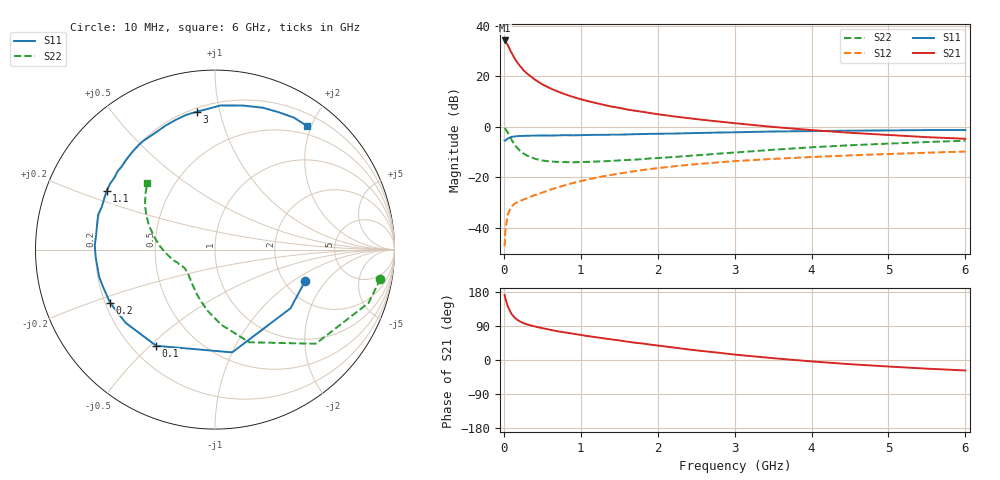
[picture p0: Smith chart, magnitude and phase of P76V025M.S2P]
! SIEMENS Small Signal Semiconductors
! BFP196
! Si NPN RF Bipolar Junction Transistor in SOT143
! VCE = 6 V  IC = 25 mA
! Common Emitter S-Parameters:  May  1996
# GHz  S  MA  R  50
!  f  S11  S21  S12  S22
! GHz  MAG  ANG  MAG  ANG  MAG  ANG  MAG  ANG
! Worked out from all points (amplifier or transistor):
!   36 points, 10 MHz to 6 GHz, reference 50 ohm
!   highest |S21| = 34.2 dB at 10 MHz (marker M1)
!   |S21| within 3 dB of that: start of sweep to 69.23 MHz
!   unconditionally stable (mu >= 1): 630.1 MHz to 4.065 GHz
!   at 250 MHz: K = 0.65, MSG = 25.8 dB, |S12| = -28.9 dB
!   at 1.4 GHz: K = 1.10, MAG = 11.6 dB, |S12| = -19.1 dB
!   at 6 GHz: K = 0.96, MSG = 2.5 dB, |S12| = -9.8 dB
!   S11 on the Smith chart (normalised r, x): 10 MHz: 2.58, -1.26; 100 MHz: 0.30, -0.52; 200 MHz: 0.22, -0.23; 1.1 GHz: 0.20, +0.24; 3 GHz: 0.22, +0.85; 6 GHz: 0.37, +1.93
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0.01  0.5318 -19.2  51.1 171.7  0.0043 81.8  0.936 -10.0
0.02  0.533 -37.8  48.81 162.6  0.0089 74.6  0.906 -19.1
0.05  0.5805 -80.5  41.47 142.3  0.018 61.0  0.768 -43.1
0.1  0.628 -121.4  29.09 121.4  0.0265 46.5  0.5504 -69.7
0.15  0.6437 -140.7  21.25 109.9  0.0305 43.3  0.4201 -85.3
0.2  0.6553 -153.2  16.65 102.7  0.0332 42.9  0.3448 -96.6
0.25  0.6571 -161.3  13.46 97.8  0.0357 43.7  0.2967 -105.5
0.3  0.6629 -166.7  11.36 94.2  0.0383 45.8  0.2687 -112.0
0.4  0.666 -176.1  8.649 88.6  0.0441 48.2  0.2325 -122.6
0.5  0.6704 178.0  6.923 84.1  0.0494 50.5  0.2138 -130.4
0.6  0.6673 172.7  5.793 79.8  0.0565 52.8  0.2052 -135.8
0.7  0.6726 167.3  4.988 75.8  0.0628 53.9  0.2006 -140.1
0.9  0.674 159.3  3.885 69.3  0.077 54.6  0.1976 -146.8
1.1  0.6866 151.6  3.192 62.9  0.0907 54.7  0.2014 -151.1
1.3  0.689 144.2  2.706 57.1  0.1048 53.3  0.2067 -155.0
1.6  0.7027 135.0  2.199 48.6  0.1248 50.8  0.2194 -159.8
2.2  0.73 117.5  1.608 33.1  0.1636 44.2  0.2505 -169.4
3  0.7747 97.6  1.174 14.3  0.208 33.9  0.3081 176.3
3.5  0.8037 87.7  0.989 4.8  0.2304 27.4  0.3489 167.6
4.5  0.8343 71.3  0.758 -11.1  0.2702 16.2  0.4285 153.3
5.5  0.8568 59.1  0.621 -22.9  0.3056 5.5  0.4968 141.3
6  0.8588 53.5  0.577 -27.6  0.322 -0.3  0.5281 135.5
